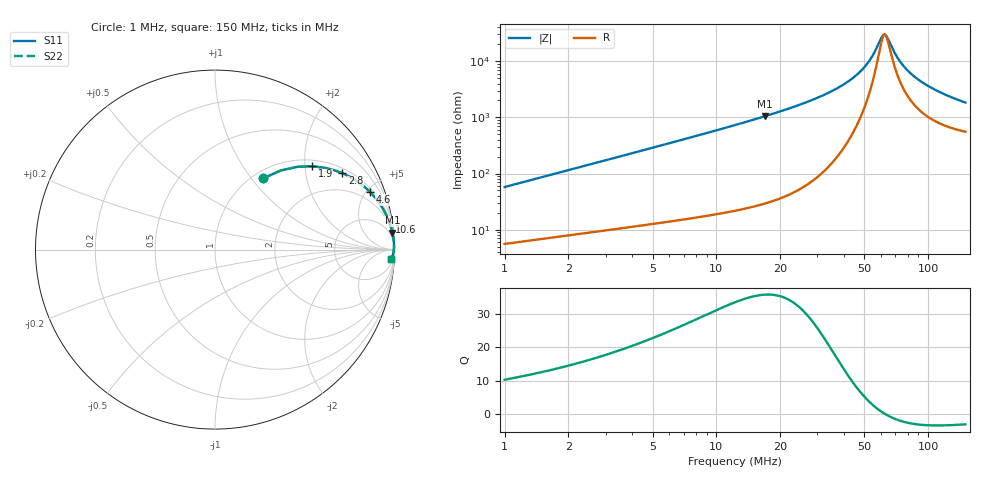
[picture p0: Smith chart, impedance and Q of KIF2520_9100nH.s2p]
!version-2
!date-12.2020
!Series
# MHz S RI R 50
!Freq ReS11 ImS11 ReS21 ImS21 ReS12 ImS12 ReS22 ImS22
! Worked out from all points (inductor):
!   498 points, 1 MHz to 150 MHz, reference 50 ohm
!   read as one part in series: L = 9.1 uH near 1.6 MHz
!   highest Q = 35.9 at 16.9 MHz (marker M1), where L = 9.82 uH
!   self-resonance near 62.5 MHz
!   S11 on the Smith chart (normalised r, x): 1 MHz: 1.11, +1.14; 1.9 MHz: 1.15, +2.17; 2.8 MHz: 1.19, +3.21; 4.6 MHz: 1.24, +5.29; 10.6 MHz: 1, +12; 150 MHz: 12, -35
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1  0.2677 0.3967  0.7323 -0.3967  0.7323 -0.3967  0.2677 0.3967
1.9  0.5402 0.4643  0.4598 -0.4643  0.4598 -0.4643  0.5402 0.4643
2.8  0.7099 0.4256  0.2901 -0.4256  0.2901 -0.4256  0.7099 0.4256
3.7  0.8068 0.3702  0.1932 -0.3702  0.1932 -0.3702  0.8068 0.3702
4.6  0.8642 0.3206  0.1358 -0.3206  0.1358 -0.3206  0.8642 0.3206
7  0.9352 0.2283  0.0648 -0.2283  0.0648 -0.2283  0.9352 0.2283
10.6  0.9704 0.1545  0.0296 -0.1545  0.0296 -0.1545  0.9704 0.1545
16.9  0.9883 0.0944  0.0117 -0.0944  0.0117 -0.0944  0.9883 0.0944
25.9  0.9951 0.0554  0.0049 -0.0554  0.0049 -0.0554  0.9951 0.0554
41.8  0.9975 0.0229  0.0025 -0.0229  0.0025 -0.0229  0.9975 0.0229
50.8  0.9974 0.0116  0.00259 -0.0116  0.00259 -0.0116  0.9974 0.0116
55  0.9972 0.00709  0.00279 -0.00709  0.00279 -0.00709  0.9972 0.00709
60.4  0.9968 0.00191  0.00316 -0.00191  0.00316 -0.00191  0.9968 0.00191
62.2  0.9967 0.000292  0.00331 -0.000292  0.00331 -0.000292  0.9967 0.000292
64  0.9965 -0.00127  0.00347 0.00127  0.00347 0.00127  0.9965 -0.00127
70.6  0.9959 -0.00665  0.00413 0.00665  0.00413 0.00665  0.9959 -0.00665
75.7  0.9953 -0.0105  0.00473 0.0105  0.00473 0.0105  0.9953 -0.0105
80.5  0.9947 -0.0139  0.00535 0.0139  0.00535 0.0139  0.9947 -0.0139
86.2  0.9939 -0.0177  0.00615 0.0177  0.00615 0.0177  0.9939 -0.0177
100.6  0.9915 -0.0264  0.00845 0.0264  0.00845 0.0264  0.9915 -0.0264
125.2  0.9868 -0.0392  0.0132 0.0392  0.0132 0.0392  0.9868 -0.0392
150  0.9812 -0.0502  0.0188 0.0502  0.0188 0.0502  0.9812 -0.0502
